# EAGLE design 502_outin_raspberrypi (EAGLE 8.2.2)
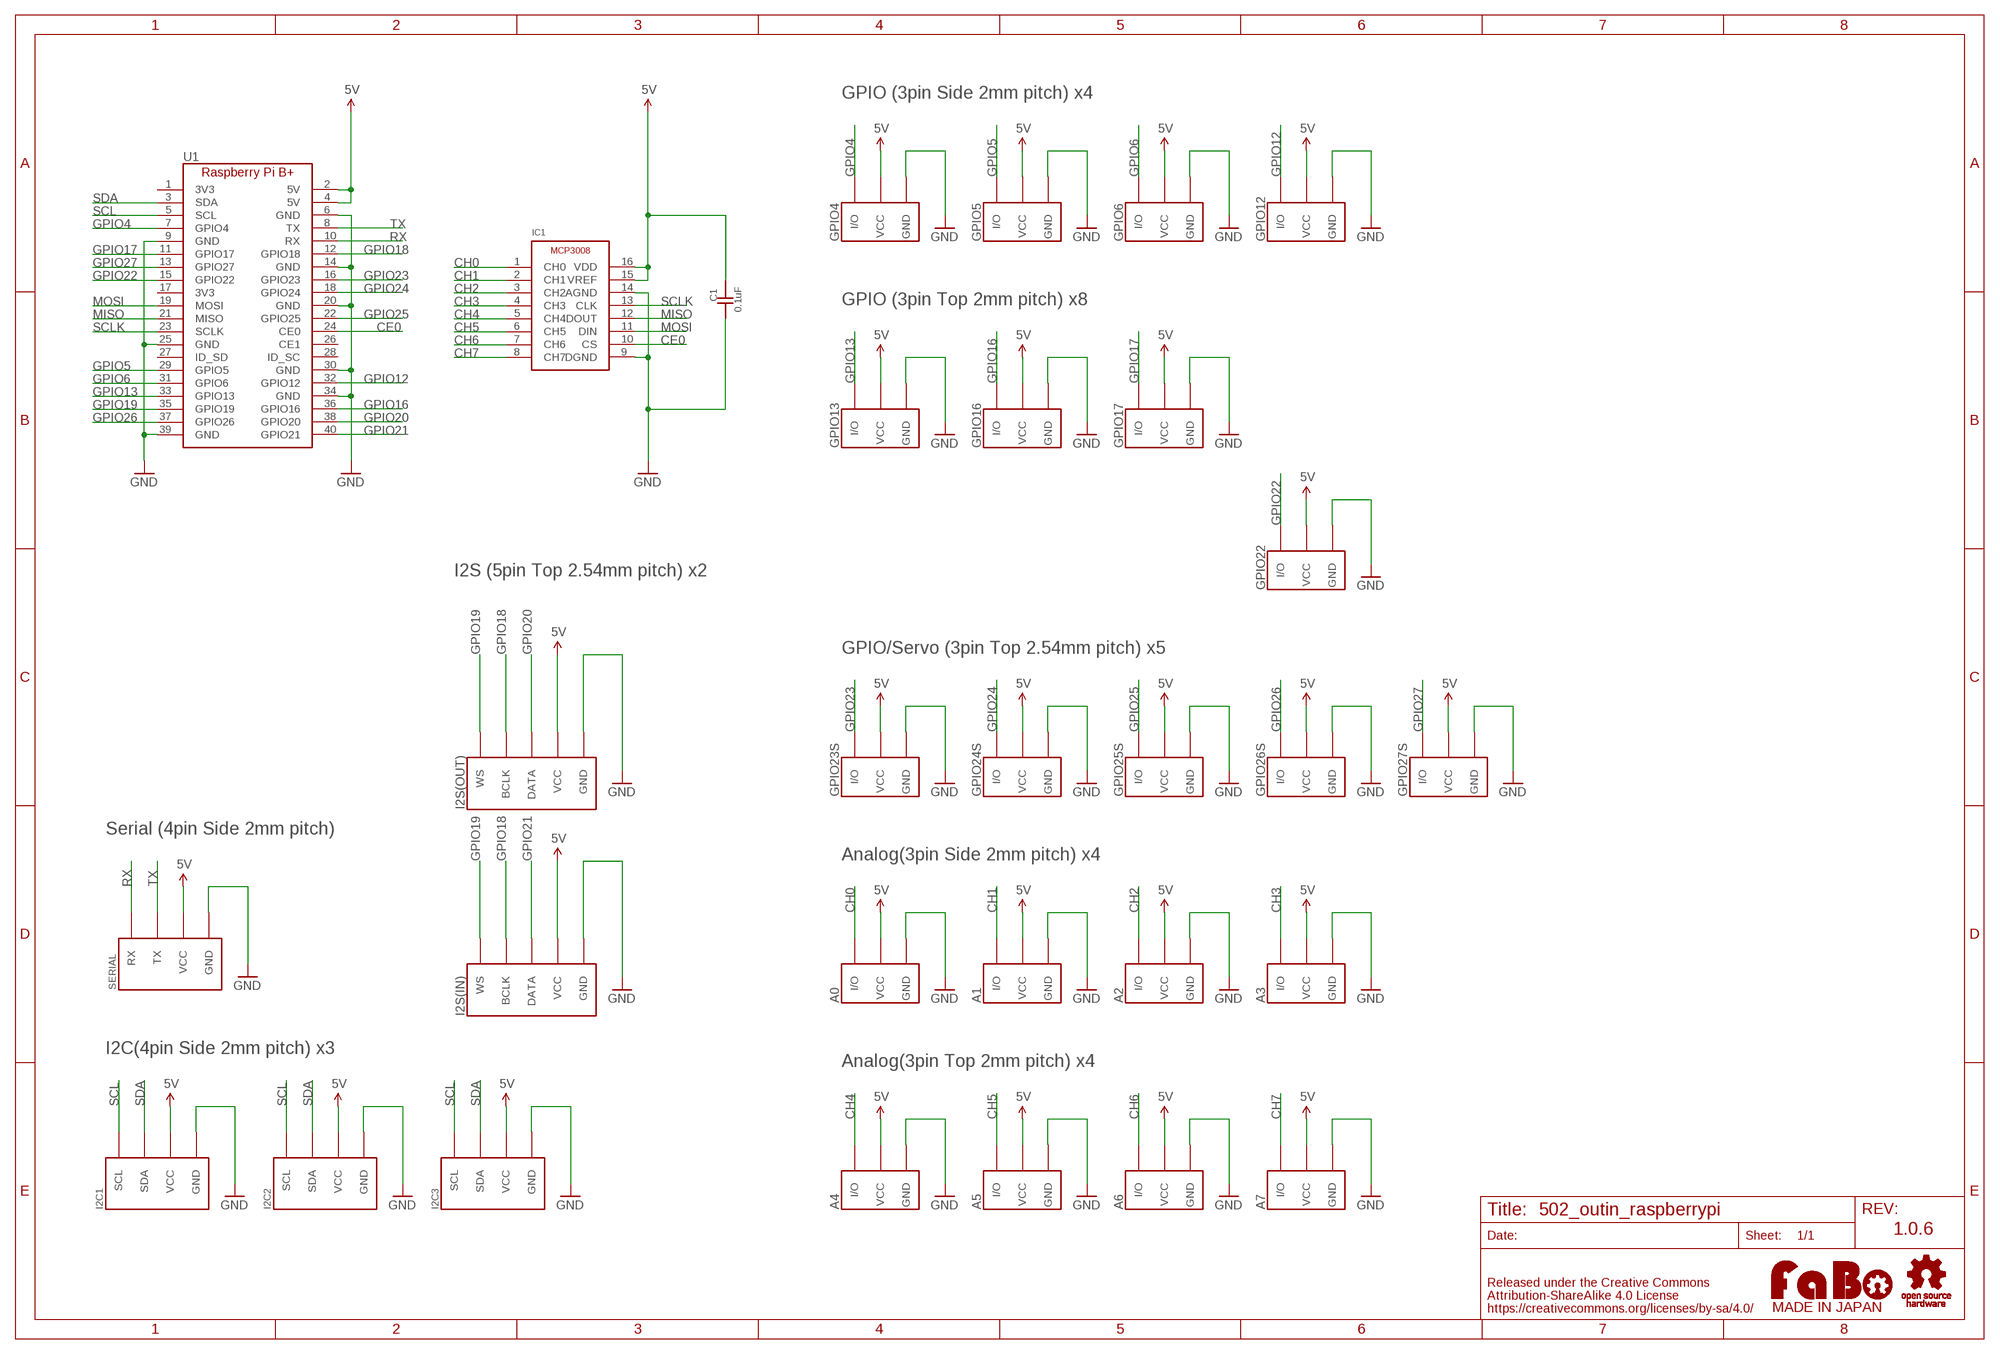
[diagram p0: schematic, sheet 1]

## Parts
A0  FABO_BRICK_3PIN-S03B-PASK-2  [FABO_BRICK_3PIN_S03B-PASK-2]
A1  FABO_BRICK_3PIN-S03B-PASK-2  [FABO_BRICK_3PIN_S03B-PASK-2]
A2  FABO_BRICK_3PIN-S03B-PASK-2  [FABO_BRICK_3PIN_S03B-PASK-2]
A3  FABO_BRICK_3PIN-S03B-PASK-2  [FABO_BRICK_3PIN_S03B-PASK-2]
A4  FABO_BRICK_3PIN-B03B-PASK-1  [FABO_BRICK_3PIN_B03B-PASK-1]
A5  FABO_BRICK_3PIN-B03B-PASK-1  [FABO_BRICK_3PIN_B03B-PASK-1]
A6  FABO_BRICK_3PIN-B03B-PASK-1  [FABO_BRICK_3PIN_B03B-PASK-1]
A7  FABO_BRICK_3PIN-B03B-PASK-1  [FABO_BRICK_3PIN_B03B-PASK-1]
C1  0.1uF  CAPACITOR-0603  [0603]
GPIO4  FABO_BRICK_3PIN-S03B-PASK-2  [FABO_BRICK_3PIN_S03B-PASK-2]
GPIO5  FABO_BRICK_3PIN-S03B-PASK-2  [FABO_BRICK_3PIN_S03B-PASK-2]
GPIO6  FABO_BRICK_3PIN-S03B-PASK-2  [FABO_BRICK_3PIN_S03B-PASK-2]
GPIO12  FABO_BRICK_3PIN-S03B-PASK-2  [FABO_BRICK_3PIN_S03B-PASK-2]
GPIO13  FABO_BRICK_3PIN-B03B-PASK-1  [FABO_BRICK_3PIN_B03B-PASK-1]
GPIO16  FABO_BRICK_3PIN-B03B-PASK-1  [FABO_BRICK_3PIN_B03B-PASK-1]
GPIO17  FABO_BRICK_3PIN-B03B-PASK-1  [FABO_BRICK_3PIN_B03B-PASK-1]
GPIO22  FABO_BRICK_3PIN-B03B-PASK-1  [FABO_BRICK_3PIN_B03B-PASK-1]
GPIO23S  FABO_BRICK_3PIN-HEADER  [FABO_BRICK_3PIN_HEADER]
GPIO24S  FABO_BRICK_3PIN-HEADER  [FABO_BRICK_3PIN_HEADER]
GPIO25S  FABO_BRICK_3PIN-HEADER  [FABO_BRICK_3PIN_HEADER]
GPIO26S  FABO_BRICK_3PIN-HEADER  [FABO_BRICK_3PIN_HEADER]
GPIO27S  FABO_BRICK_3PIN-HEADER  [FABO_BRICK_3PIN_HEADER]
I2C1  FABO_BRICK_I2C-S04B-PASK-2  [FABO_BRICK_I2C_S04B-PASK-2]
I2C2  FABO_BRICK_I2C-S04B-PASK-2  [FABO_BRICK_I2C_S04B-PASK-2]
I2C3  FABO_BRICK_I2C-S04B-PASK-2  [FABO_BRICK_I2C_S04B-PASK-2]
I2S(IN)  FABO_BRICK_I2SLONG  [FABO_BRICK_I2S_S05B-PASK-2_LONG]
I2S(OUT)  FABO_BRICK_I2SLONG  [FABO_BRICK_I2S_S05B-PASK-2_LONG]
IC1  MICROCHIP-MCP3008  [MICROCHIP-MCP3008]
SERIAL  FABO_BRICK_SERIAL-S04B-PASK-2  [FABO_BRICK_SERIAL_S04B-PASK-2]
U1  RASPBERRY_PI_B+  [RASPBERRY_PI_B+]
U$4  LOGO_OSHW-T_M_BOTTOM  [LOGO_OSHW_T_MS_BOTTOM]
U$14  LOGO_FABO-M  [LOGO_FABO_MS]

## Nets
5V: A0.VCC A1.VCC A2.VCC A3.VCC A4.VCC A5.VCC A6.VCC A7.VCC C1.2 GPIO4.VCC GPIO5.VCC GPIO6.VCC GPIO12.VCC GPIO13.VCC GPIO16.VCC GPIO17.VCC GPIO22.VCC GPIO23S.VCC GPIO24S.VCC GPIO25S.VCC GPIO26S.VCC GPIO27S.VCC I2C1.VCC I2C2.VCC I2C3.VCC I2S(IN).VCC I2S(OUT).VCC IC1.15(VREF) IC1.16(VDD) SERIAL.VCC U1.2(5V) U1.4(5V)
CE0: IC1.10(CS) U1.24(CE0)
CH0: A0.I/O IC1.1(CH0)
CH1: A1.I/O IC1.2(CH1)
CH2: A2.I/O IC1.3(CH2)
CH3: A3.I/O IC1.4(CH3)
CH4: A4.I/O IC1.5(CH4)
CH5: A5.I/O IC1.6(CH5)
CH6: A6.I/O IC1.7(CH6)
CH7: A7.I/O IC1.8(CH7)
GND: A0.GND A1.GND A2.GND A3.GND A4.GND A5.GND A6.GND A7.GND C1.1 GPIO4.GND GPIO5.GND GPIO6.GND GPIO12.GND GPIO13.GND GPIO16.GND GPIO17.GND GPIO22.GND GPIO23S.GND GPIO24S.GND GPIO25S.GND GPIO26S.GND GPIO27S.GND I2C1.GND I2C2.GND I2C3.GND I2S(IN).GND I2S(OUT).GND IC1.9(DGND) IC1.14(AGND) SERIAL.GND U1.6(GND) U1.9(GND) U1.14(GND) U1.20(GND) U1.25(GND) U1.30(GND) U1.34(GND) U1.39(GND)
GPIO4: GPIO4.I/O U1.7(GPIO4)
GPIO5: GPIO5.I/O U1.29(GPIO5)
GPIO6: GPIO6.I/O U1.31(GPIO6)
GPIO12: GPIO12.I/O U1.32(GPIO12)
GPIO13: GPIO13.I/O U1.33(GPIO13)
GPIO16: GPIO16.I/O U1.36(GPIO16)
GPIO17: GPIO17.I/O U1.11(GPIO17)
GPIO18: I2S(IN).BCLK I2S(OUT).BCLK U1.12(GPIO18)
GPIO19: I2S(IN).WS I2S(OUT).WS U1.35(GPIO19)
GPIO20: I2S(OUT).DATA U1.38(GPIO20)
GPIO21: I2S(IN).DATA U1.40(GPIO21)
GPIO22: GPIO22.I/O U1.15(GPIO22)
GPIO23: GPIO23S.I/O U1.16(GPIO23)
GPIO24: GPIO24S.I/O U1.18(GPIO24)
GPIO25: GPIO25S.I/O U1.22(GPIO25)
GPIO26: GPIO26S.I/O U1.37(GPIO26)
GPIO27: GPIO27S.I/O U1.13(GPIO27)
MISO: IC1.12(DOUT) U1.21(MISO)
MOSI: IC1.11(DIN) U1.19(MOSI)
RX: SERIAL.RX U1.10(RX)
SCL: I2C1.SCL I2C2.SCL I2C3.SCL U1.5(SCL)
SCLK: IC1.13(CLK) U1.23(SCLK)
SDA: I2C1.SDA I2C2.SDA I2C3.SDA U1.3(SDA)
TX: SERIAL.TX U1.8(TX)
Unconnected: U1.1(3V3) U1.17(3V3) U1.26(CE1) U1.27(ID_SD) U1.28(ID_SC)

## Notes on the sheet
- GPIO (3pin Side 2mm pitch) x4
- GPIO (3pin Top 2mm pitch) x8
- I2S (5pin Top 2.54mm pitch) x2
- GPIO/Servo (3pin Top 2.54mm pitch) x5
- Serial (4pin Side 2mm pitch)
- Analog(3pin Side 2mm pitch) x4
- I2C(4pin Side 2mm pitch) x3
- Analog(3pin Top 2mm pitch) x4
- 1.0.6

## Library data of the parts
A0 A1-A7 GPIO4-GPIO6 GPIO12 GPIO13 GPIO16 GPIO17 GPIO22 GPIO23S GPIO24S GPIO25S GPIO26S GPIO27S = FaBo-Template:FABO_BRICK_3PIN: FaBo Brick 3pin
C1 = FaBo-Capacitor:CAPACITOR: CAPACITOR
I2C1-I2C3 = FaBo-Template:FABO_BRICK_I2C: FaBo Brick I2C
I2S(IN) I2S(OUT) = FaBo-Template:FABO_BRICK_I2S
IC1 = FaBo-ADC:MICROCHIP-MCP3008
SERIAL = FaBo-Template:FABO_BRICK_SERIAL: FaBo Brick Serial
U1 = FaBo-Boards:RASPBERRY_PI_B+
U$4 = FaBo-etc:LOGO_OSHW
U$14 = FaBo-etc:LOGO_FABO

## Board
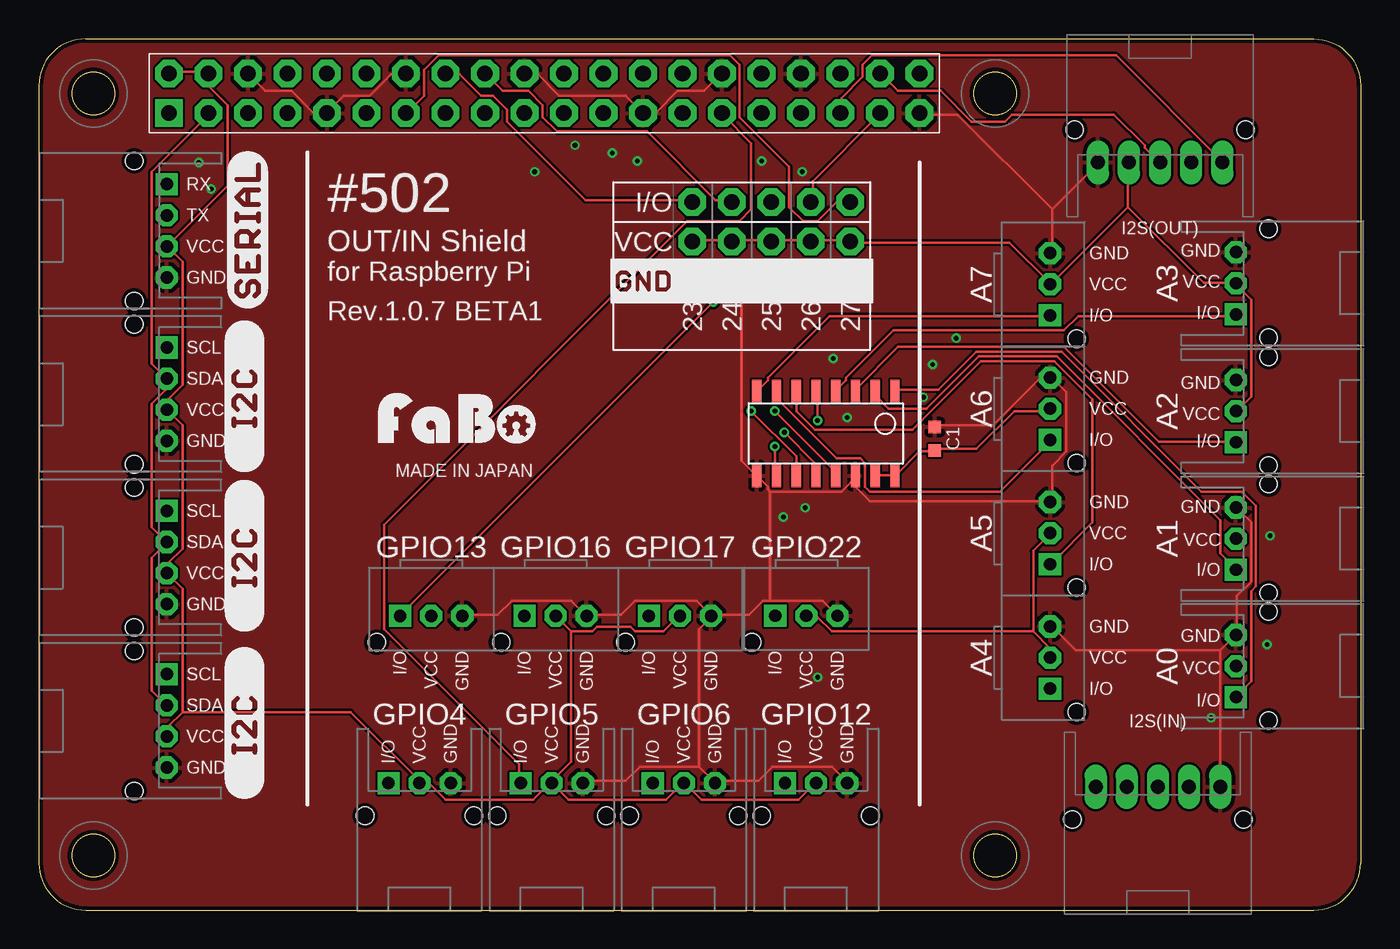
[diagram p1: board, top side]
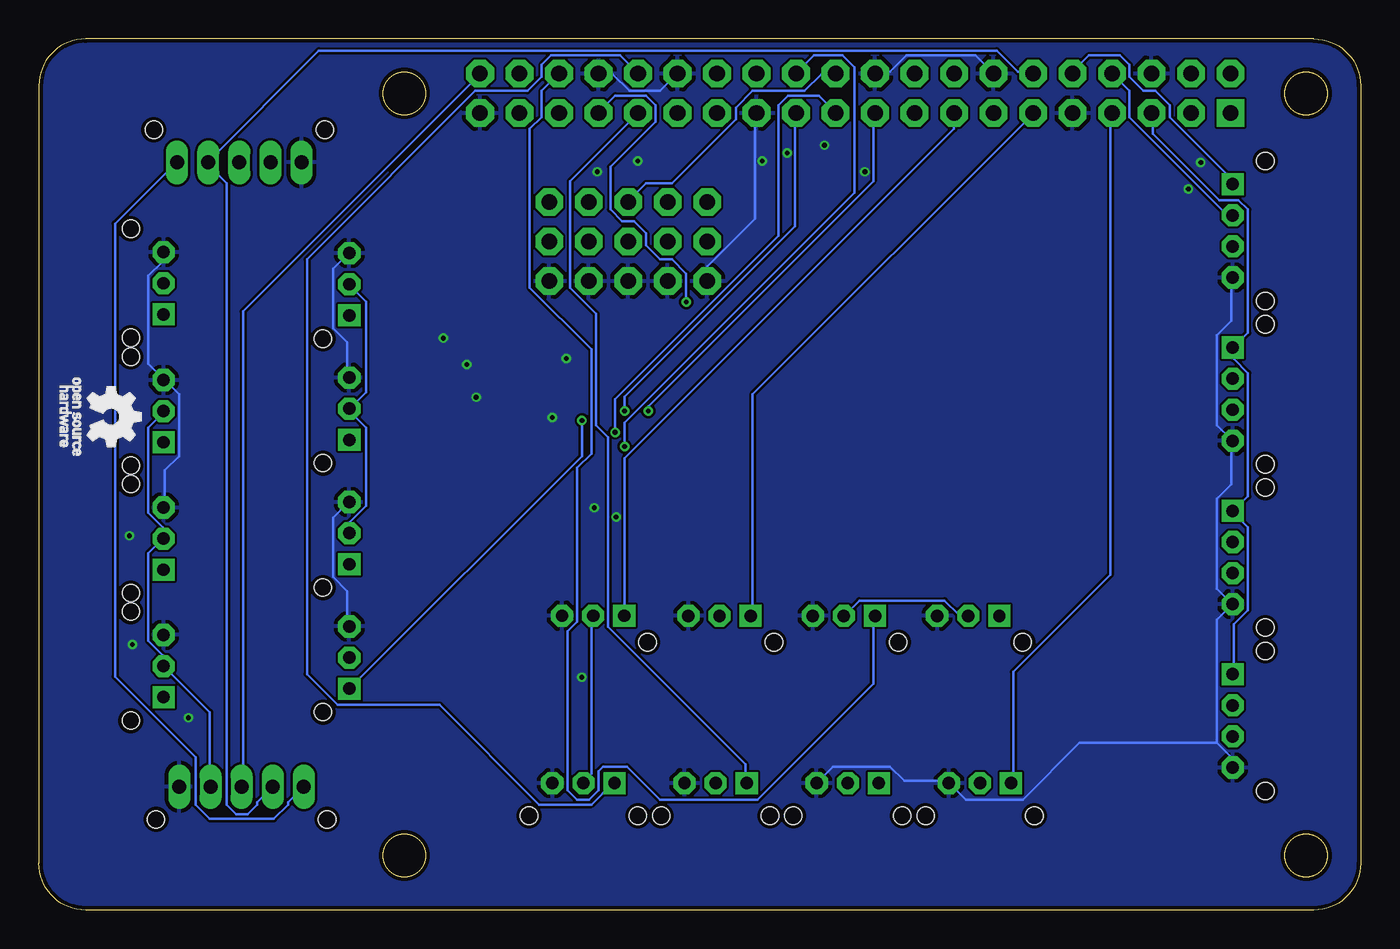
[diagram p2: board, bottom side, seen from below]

Size 85 x 56 mm. Coordinates in mm from the lower left corner, seen from the top.
Copper layers (1*16): Top 0.035mm / dielectric 1.5mm / Bottom 0.035mm
Design rules "Elecrow_2-layer_eagle_rule": minimum track width 6mil, minimum drill 12mil, track to track 6mil, track to pad 6mil, pad to pad 6mil, via to via 6mil, smd to smd 0mil, copper to edge 10mil, drill to drill 10mil, minimum pad ring 10mil, minimum via ring 6mil, stop-mask expansion 2mil, vias tented up to drill 100mil, thermal gap 10mil

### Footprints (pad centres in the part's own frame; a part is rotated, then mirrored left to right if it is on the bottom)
FABO_BRICK_3PIN_S03B-PASK-2 = drill 0.8 pad 1.422 octagon: GND -2,0; VCC 0,0 | drill 0.8 pad 1.422 square: I/O 2,0 | hole 1.1: 3.5,2.1; -3.5,2.1
FABO_BRICK_3PIN_B03B-PASK-1 = drill 0.8 pad 1.422 octagon: GND -2,0; VCC 0,0 | drill 0.8 pad 1.422 square: I/O 2,0 | hole 1.1: 3.5,1.7
0603 = smd 0.8 x 0.8: 1 -0.75,0; 2 0.75,0
FABO_BRICK_3PIN_HEADER = drill 1 pad 1.778 octagon: GND -2.54,0; I/O 2.54,0; VCC 0,0
FABO_BRICK_I2C_S04B-PASK-2 = drill 0.8 pad 1.422 octagon: GND -3,0; SDA 1,0; VCC -1,0 | drill 0.8 pad 1.422 square: SCL 3,0 | hole 1.1: 4.5,2.1; -4.5,2.1
FABO_BRICK_I2S_S05B-PASK-2_LONG = drill 0.9 pad 1.422 long: BCLK 3,0; DATA 1,0; GND -3,0; VCC -1,0; WS 5,0 | hole 1.1: 6.5,2.1; -4.5,2.1
MICROCHIP-MCP3008 = smd 0.6 x 1.5: 1 -4.445,-2.7; 2 -3.175,-2.7; 3 -1.905,-2.7; 4 -0.635,-2.7; 5 0.635,-2.7; 6 1.905,-2.7; 7 3.175,-2.7; 8 4.445,-2.7; 9 4.445,2.7; 10 3.175,2.7; 11 1.905,2.7; 12 0.635,2.7; 13 -0.635,2.7; 14 -1.905,2.7; 15 -3.175,2.7; 16 -4.445,2.7
FABO_BRICK_SERIAL_S04B-PASK-2 = drill 0.8 pad 1.422 octagon: GND -3,0; TX 1,0; VCC -1,0 | drill 0.8 pad 1.422 square: RX 3,0 | hole 1.1: 4.5,2.1; -4.5,2.1
RASPBERRY_PI_B+ = drill 1 pad 1.778 square: 1 0,-2.54 | drill 1 pad 1.778 octagon: 2 0,0; 3 2.54,-2.54; 4 2.54,0; 5 5.08,-2.54; 6 5.08,0; 7 7.62,-2.54; 8 7.62,0; 9 10.16,-2.54; 10 10.16,0; 11 12.7,-2.54; 12 12.7,0; 13 15.24,-2.54; 14 15.24,0; 15 17.78,-2.54; 16 17.78,0; 17 20.32,-2.54; 18 20.32,0; 19 22.86,-2.54; 20 22.86,0; 21 25.4,-2.54; 22 25.4,0; 23 27.94,-2.54; 24 27.94,0; 25 30.48,-2.54; 26 30.48,0; 27 33.02,-2.54; 28 33.02,0; 29 35.56,-2.54; 30 35.56,0; 31 38.1,-2.54; 32 38.1,0; 33 40.64,-2.54; 34 40.64,0; 35 43.18,-2.54; 36 43.18,0; 37 45.72,-2.54; 38 45.72,0; 39 48.26,-2.54; 40 48.26,0

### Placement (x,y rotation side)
A0  76.98,15.68 270 top
A1  76.98,23.88 270 top
A2  76.98,32.07 270 top
A3  76.98,40.29 270 top
A4  65.03,16.23 270 top
A5  65.03,24.23 270 top
A6  65.03,32.23 270 top
A7  65.03,40.23 270 top
C1  57.62,30.3 270 top
GPIO4  24.48,8.16 180 top
GPIO5  32.98,8.16 180 top
GPIO6  41.48,8.16 180 top
GPIO12  49.98,8.16 180 top
GPIO13  25.23,18.91 180 top
GPIO16  33.23,18.91 180 top
GPIO17  41.23,18.91 180 top
GPIO22  49.36,18.92 180 top
GPIO23S  42.02,42.98 90 top
GPIO24S  44.56,42.98 90 top
GPIO25S  47.1,42.98 90 top
GPIO26S  49.64,42.98 90 top
GPIO27S  52.18,42.98 90 top
I2C1  8.23,33.16 90 top
I2C2  8.23,22.66 90 top
I2C3  8.23,12.16 90 top
I2S(IN)  72.96,7.92 180 top
I2S(OUT)  71.11,48.06 0 top
IC1  50.61,30.63 180 top
SERIAL  8.23,43.66 90 top
U1  8.37,53.77 0 top
U$2  [LOGO_SILK_I2C]  14.48,17.91 90 top
U$3  [LOGO_SILK_SERIAL2]  14.73,38.66 90 top
U$4  80.38,31.7 90 top
U$5  [LOGO_SILK_I2C]  14.48,7.16 90 top
U$6  [LOGO_SILK_I2C]  14.48,28.16 90 top
U$7  [LOGO_SILK_GND]  36.95,39.17 0 top
U$14  26.89,29.61 0 top

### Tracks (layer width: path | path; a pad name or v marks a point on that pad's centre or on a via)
5V
  Top 0.152: 9.23,12.72 8.32,11.81 8.32,11.2 I2C3.VCC | 9.23,12.72 9.23,20.65 8.32,21.56 I2C2.VCC 8.32,21.72 8.32,22.33 9.23,23.24 9.23,31.16 8.32,32.08 I2C1.VCC 8.32,32.23 8.32,32.84 9.23,33.76 9.23,41.68 8.32,42.59 SERIAL.VCC 8.32,42.75 12.13,46.56 12.13,51.74 10.91,52.96 U1.4 10.91,53.87 8.47,53.87 U1.2 | 34.23,17.91 35.6,17.91 35.9,18.21 38.04,18.21 38.34,17.91 40.17,17.91 41.08,18.82 GPIO17.VCC | 34.23,17.91 33.31,18.82 GPIO16.VCC | GPIO5.VCC 32.86,8.15 31.79,7.09 26.15,7.09 25.08,8.15 24.63,8.15 GPIO4.VCC 24.47,8.3 20.05,12.72 9.23,12.72 | GPIO5.VCC 33.01,8.15 34.07,7.09 40.32,7.09 41.39,8.15 GPIO6.VCC 41.54,8.15 42.61,7.09 48.86,7.09 49.92,8.15 GPIO12.VCC | 34.23,17.91 34.23,9.52 33.01,8.3 GPIO5.VCC | A2.VCC 77.05,32.08 77.97,32.99 77.97,39.24 77.05,40.16 A3.VCC 76.9,40.31 74.92,40.31 70.04,45.19 | GPIO23S.VCC 42.15,43.05 44.44,43.05 GPIO24S.VCC 44.59,43.05 47.03,43.05 GPIO25S.VCC 47.18,43.05 49.62,43.05 GPIO26S.VCC 49.77,43.05 52.06,43.05 GPIO27S.VCC 52.21,42.9 62.42,42.9 65.01,40.31 A7.VCC 65.16,40.31 70.04,45.19 | 63.95,17.91 65.01,16.84 65.01,16.23 A4.VCC | 63.95,17.91 63.95,23.09 65.01,24.15 A5.VCC | IC1.15 53.89,27.96 54.95,27.96 IC1.16 55.11,27.96 56.63,29.49 57.54,29.49 C1.2 57.7,29.64 60.29,29.64 62.73,32.08 65.01,32.08 A6.VCC | 70.04,45.19 70.04,47.93 I2S(OUT).VCC | 63.95,17.91 50.99,17.91 50.08,18.82 49.47,18.82 GPIO22.VCC
  Bottom 0.152: GPIO13.VCC 25.24,18.97 25.84,18.97 26.76,19.89 32.25,19.89 33.16,18.97 GPIO16.VCC | GPIO22.VCC 49.47,18.82 49.47,8.76 49.92,8.3 GPIO12.VCC | I2S(IN).VCC 74,8 74,12.72 76.9,15.62 A0.VCC 77.05,15.77 77.05,16.38 77.97,17.3 77.97,22.93 77.05,23.85 A1.VCC 77.05,24 77.05,24.61 77.97,25.53 77.97,31.01 77.05,31.93 A2.VCC | A7.VCC 65.01,40.16 63.95,39.09 63.95,33.3 65.01,32.23 A6.VCC 65.01,32.08 63.95,31.01 63.95,25.98 65.01,24.92 65.01,24.31 A5.VCC
CE0  (via drill 0.3)
  Top 0.152: v47.33,29.79 47.33,27.96 IC1.10
  Bottom 0.152: v47.33,29.79 47.33,31.32 32.55,46.1 32.55,54.18 33.31,54.94 35.14,54.94 U1.24
CH0
  Top 0.152: IC1.1 55.11,33.45 57.85,33.45 60.29,35.89 65.77,35.89 74.77,26.9 77.36,26.9 78.27,25.98 78.27,20.8 77.97,20.5 77.97,14.71 77.05,13.79 A0.I/O
CH1
  Top 0.152: IC1.2 53.89,33.3 53.89,32.99 54.65,32.23 57.09,32.23 60.44,35.58 65.47,35.58 75.98,25.07 75.98,22.93 76.9,22.02 A1.I/O
CH2
  Top 0.152: IC1.3 52.51,33.45 55.26,36.19 65.93,36.19 72.02,30.1 76.9,30.1 A2.I/O
CH3
  Top 0.152: IC1.4 51.3,33.45 51.91,34.06 51.91,34.21 54.95,37.26 65.93,37.26 66.84,38.17 76.9,38.17 A3.I/O
CH4  (via drill 0.3)
  Top 0.152: v50.08,31.47 50.08,33.3 IC1.5
  Bottom 0.152: v50.08,31.47 50.08,29.18 65.01,14.25 A4.I/O
CH5
  Top 0.152: IC1.6 48.7,32.08 49.92,30.86 56.17,30.86 60.59,35.28 65.32,35.28 67.76,32.84 67.76,24.92 65.16,22.33 A5.I/O
CH6
  Top 0.152: IC1.7 47.49,33.3 47.49,32.84 51.3,29.03 52.82,29.03 53.12,28.73 53.12,27.2 53.43,26.9 61.81,26.9 65.01,30.1 A6.I/O
CH7
  Top 0.152: IC1.8 46.27,33.45 46.88,34.06 46.88,34.21 50.84,38.17 65.01,38.17 A7.I/O
GND  (via drill 0.3)
  Top 0.152: 75.98,16.69 75.98,8 I2S(IN).GND | 75.98,16.69 76.9,17.6 A0.GND 77.05,17.75 77.05,20.19 77.97,21.11 77.97,24.92 77.05,25.83 A1.GND | C1.1 57.7,31.16 61.35,31.16 64.4,34.21 65.01,34.21 A6.GND 65.16,34.21 66.08,33.3 66.08,29.49 65.16,28.57 65.16,26.29 A5.GND 65.01,26.29 53.43,26.29 52.21,27.51 | 65.16,45.03 65.16,42.29 A7.GND | 65.16,45.03 68.06,47.93 I2S(OUT).GND | 65.16,45.03 59.07,51.13 56.63,51.13 U1.39 | 75.98,16.69 66.69,16.69 65.16,18.21 A4.GND | 18.53,51.28 17.62,51.28 16.24,52.65 14.57,52.65 U1.6 | 18.53,51.28 19.6,52.35 21.27,52.35 22.64,53.72 23.56,53.72 U1.14 | 18.53,51.28 U1.9 | GPIO23S.GND 42.15,40.46 44.44,40.46 GPIO24S.GND | GPIO27S.GND 52.06,40.46 49.77,40.46 GPIO26S.GND 49.62,40.46 47.18,40.46 GPIO25S.GND 47.03,40.46 45.2,40.46 | 45.2,40.46 44.59,40.46 GPIO24S.GND | U1.30 43.83,53.72 42.76,52.65 41.08,52.65 39.71,51.28 38.95,51.28 U1.25 37.73,52.35 33.46,52.35 32.09,53.72 31.33,53.72 U1.20 | GPIO12.GND 51.91,8.3 50.99,9.22 47.18,9.22 46.27,8.3 43.52,8.3 GPIO6.GND 43.37,8.3 42.46,9.22 | 42.46,9.22 38.65,9.22 37.73,8.3 34.99,8.3 GPIO5.GND | GPIO13.GND 27.37,18.97 29.5,18.97 30.42,19.89 34.23,19.89 35.14,18.97 GPIO16.GND 35.29,18.97 37.43,18.97 38.34,19.89 42.3,19.89 43.22,18.97 GPIO17.GND | 47.03,26.9 46.88,27.05 46.88,27.2 46.27,27.81 IC1.9 46.11,27.96 45.2,28.88 45.2,40.46 | 47.03,26.9 51.6,26.9 52.21,27.51 | 52.21,27.51 52.51,27.81 IC1.14 | 47.03,19.89 50.38,19.89 51.3,18.97 GPIO22.GND | 47.03,19.89 46.57,19.89 45.66,18.97 43.37,18.97 GPIO17.GND | 47.03,19.89 47.03,26.9 | 42.46,9.22 42.46,18.06 43.22,18.82 GPIO17.GND | 45.2,40.46 GPIO24S.GND
  Bottom 0.152: A1.GND 76.9,25.98 76.9,28.27 75.98,29.18 75.98,33.15 76.9,34.06 A2.GND 77.05,34.21 77.97,35.13 77.97,40.77 77.05,41.68 77.05,42.29 A3.GND | A4.GND 65.16,18.36 65.16,20.5 66.08,21.41 66.08,25.22 65.16,26.14 A5.GND | A6.GND 65.16,34.36 65.16,36.5 66.08,37.41 66.08,41.22 65.16,42.14 A7.GND | U1.14 24.78,54.94 29.2,54.94 30.27,53.87 31.18,53.87 U1.20 | U1.30 45.05,52.65 47.03,52.65 48.1,53.72 49.01,53.72 U1.34 | GPIO23S.GND 42,40.46 42,41.38 38.95,44.42 38.95,51.13 U1.25 | 9.23,10.74 8.32,9.83 8.32,9.22 I2C3.GND | 9.23,10.74 9.23,18.67 8.32,19.58 I2C2.GND 8.32,19.73 9.23,20.65 9.23,26.44 8.32,27.35 8.32,30.1 I2C1.GND 8.32,30.25 9.23,31.16 9.23,36.96 8.32,37.87 8.32,40.61 SERIAL.GND | GPIO5.GND 34.84,8.3 33.92,9.22 30.27,9.22 29.35,8.3 26.61,8.3 GPIO4.GND 26.45,8.15 25.39,7.09 21.73,7.09 18.07,10.74 9.23,10.74
  other vias: 34.48,49.16 38.48,48.16 46.48,48.16 49.08,47.46 51.08,35.46 57.48,35.06 51.98,31.66 49.28,25.86 50.08,14.96 10.28,48.06 11.08,46.36 31.88,47.46 36.88,48.66 58.98,36.76 56.88,32.96 47.88,25.26 75.38,12.36 79.18,24.06 78.98,17.06
  pour Bottom: -0.52,-0.84 85.48,-0.84 85.48,56.16 -0.52,56.16
  pour Top: -0.52,-0.84 85.48,-0.84 85.48,56.16 -0.52,56.16
GPIO4
  Bottom 0.152: GPIO4.I/O 22.34,8.3 22.34,15.31 16.09,21.56 16.09,51.13 U1.7
GPIO5
  Top 0.152: GPIO5.I/O 30.87,8.3 30.87,9.37 22.19,18.06 22.19,24.76 41.7,44.27 45.05,44.27 45.81,45.03 45.81,49.3 43.98,51.13 U1.29
GPIO6
  Bottom 0.152: U1.31 50.84,46.86 50.84,40 49.16,38.33 49.16,31.16 48.4,30.4 48.4,18.21 39.56,9.37 39.56,8.3 GPIO6.I/O
GPIO12
  Bottom 0.152: U1.32 47.64,54.94 52.06,54.94 52.67,54.33 52.67,53.57 53.58,52.65 56.93,52.65 67.76,41.83 67.76,15.16 65.77,13.18 59.22,13.18 52.82,6.78 49.47,6.78 48.1,8.15 GPIO12.I/O
GPIO13  (via drill 0.3)
  Top 0.152: v43.37,39.09 23.25,18.97 GPIO13.I/O
  Bottom 0.152: v43.37,39.09 43.37,40.92 44.29,41.83 45.05,41.83 45.96,42.75 45.96,43.51 46.72,44.27 47.49,44.27 48.25,45.03 48.25,47.78 45.35,50.67 45.35,51.74 45.96,52.35 47.94,52.35 49.01,51.28 U1.33
GPIO16
  Bottom 0.152: U1.36 52.67,52.65 52.67,50.98 53.43,50.21 53.43,40 49.47,36.04 49.47,29.34 50.38,28.42 50.38,18.52 50.99,17.91 50.99,7.69 50.38,7.09 49.62,7.09 49.01,7.69 49.01,8.91 48.7,9.22 47.18,9.22 45.05,7.09 38.8,7.09 31.33,14.55 31.33,18.82 GPIO16.I/O
GPIO17
  Bottom 0.152: GPIO17.I/O 39.1,18.97 39.1,33.15 21.12,51.13 U1.11
GPIO18
  Bottom 0.152: I2S(IN).BCLK 70.04,7.85 70.96,6.93 70.96,6.78 71.56,6.17 72.33,6.17 72.94,6.78 72.94,46.71 74.16,47.93 I2S(OUT).BCLK 74.16,48.08 66.99,55.24 23.41,55.24 22.03,53.87 21.12,53.87 U1.12
GPIO19
  Top 0.152: U1.35 51.6,51.28 51.6,52.2 52.97,53.57 52.97,54.33 53.58,54.94 69.28,54.94 76.14,48.08 I2S(OUT).WS
  Bottom 0.152: I2S(IN).WS 68.06,7.85 68.97,6.93 68.97,6.78 69.89,5.87 74,5.87 74.92,6.78 74.92,9.83 80.1,15.01 80.1,44.12 76.14,48.08 I2S(OUT).WS
GPIO20
  Top 0.152: I2S(OUT).DATA 72.02,48.08 71.11,49 71.11,49.15 69.13,51.13 62.57,51.13 62.12,50.67 59.98,50.67 58,52.65 55.26,52.65 54.19,53.72 U1.38
GPIO21
  Bottom 0.152: I2S(IN).DATA 71.87,8 71.87,38.48 56.63,53.72 U1.40
GPIO22
  Bottom 0.152: U1.15 26.15,50.21 47.33,29.03 47.33,18.97 GPIO22.I/O
GPIO23
  Top 0.152: U1.16 26.15,53.72 27.06,53.72 28.44,52.35 29.2,52.35 30.11,51.43 30.11,50.67 35.14,45.64 42,45.64 GPIO23S.I/O
GPIO24
  Top 0.152: U1.18 29.81,52.65 31.48,52.65 32.4,51.74 32.4,50.98 33.31,50.06 39.1,50.06 43.52,45.64 44.44,45.64 GPIO24S.I/O
GPIO25
  Bottom 0.152: U1.22 33.77,53.72 34.68,53.72 35.75,52.65 39.1,52.65 40.17,51.59 40.17,50.82 44.29,46.71 45.96,46.71 47.03,45.64 GPIO25S.I/O
GPIO26
  Top 0.152: GPIO26S.I/O 49.77,45.64 49.77,46.86 54.04,51.13 U1.37
GPIO27
  Top 0.152: GPIO27S.I/O 52.06,45.49 51.3,45.49 50.08,44.27 49.16,44.27 48.25,45.19 48.25,47.78 45.05,50.98 45.05,54.33 44.44,54.94 25.69,54.94 24.78,54.02 24.78,52.35 23.71,51.28 U1.13
MISO  (via drill 0.3)
  Top 0.152: v47.94,30.71 49.92,28.73 49.92,27.96 IC1.12
  Bottom 0.152: v47.94,30.71 47.94,32.84 37.43,43.36 37.43,51.74 36.82,52.35 34.84,52.35 33.77,51.28 U1.21
MOSI  (via drill 0.3)
  Top 0.152: IC1.11 48.7,29.18 v45.81,32.08
  Bottom 0.152: v45.81,32.08 45.81,32.38 31.33,46.86 31.33,51.13 U1.19
RX
  Bottom 0.152: SERIAL.RX 8.32,46.71 8.32,47.01 12.28,50.98 12.28,51.74 13.2,52.65 13.96,52.65 14.87,53.57 14.87,54.33 15.48,54.94 17.46,54.94 18.53,53.87 U1.10
SCL
  Bottom 0.152: I2C3.SCL 8.17,15.16 8.17,18.36 7.25,19.28 7.25,24.61 8.17,25.53 I2C2.SCL 8.17,25.68 7.25,26.59 7.25,34.52 8.17,35.43 8.17,36.04 I2C1.SCL 8.17,36.19 7.25,37.11 7.25,45.03 7.86,45.64 9.08,45.64 13.35,49.91 13.35,51.13 U1.5
SCLK  (via drill 0.3)
  Top 0.152: v47.33,32.08 51.14,28.27 51.14,27.96 IC1.13
  Bottom 0.152: v47.33,32.08 47.33,32.99 36.36,43.97 36.36,51.13 U1.23
SDA
  Top 0.152: I2C3.SDA 8.17,13.18 7.25,14.1 7.25,22.63 8.17,23.54 I2C2.SDA 8.17,23.7 7.25,24.61 7.25,32.54 8.17,33.45 8.17,34.06 I2C1.SDA 8.17,34.21 7.25,35.13 7.25,47.47 10.91,51.13 U1.3
TX
  Bottom 0.152: U1.8 14.87,52.65 14.87,50.98 8.62,44.73 8.32,44.73 SERIAL.TX

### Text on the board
tPlace: RX | TX | #502 | I/O | VCC | VCC | OUT/IN Shield | GND | GND | GND | for Raspberry Pi | VCC | VCC | 23 | 24 | 25 | 26 | 27 | Rev.1.0.7 BETA1 | I/O | I/O | SCL | SDA | GND | GND | VCC | VCC | VCC | GND | I/O | I/O | MADE IN JAPAN | GND | GND | SCL | VCC | VCC | SDA | I/O | I/O | VCC | GND | GND | I/O | VCC | GND | I/O | VCC | GND | I/O | VCC | GND | I/O | VCC | GND | GND | VCC | SCL | VCC | I/O | SDA | I/O | VCC | GND | I/O | VCC | GND | I/O | VCC | GND | I/O | VCC | GND | I/O | VCC | GND

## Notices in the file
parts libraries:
FaBo-etc: Released under the Creative Commons Attribution-ShareAlike 4.0 License
https://creativecommons.org/licenses/by-sa/4.0
FaBo-etc: Released under the Creative Commons
